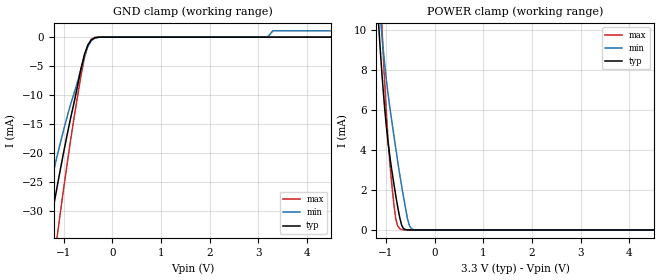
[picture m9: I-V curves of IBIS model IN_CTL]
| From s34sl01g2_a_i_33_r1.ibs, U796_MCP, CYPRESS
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|Driver/receiver models for NAND component of MCP
|   Model IN_CTL
[Model]  IN_CTL
Model_type Input
Vinl =   0.6600V | Vinl = Vio*0.3
Vinh =   2.6400V | Vinh = Vio*0.8
C_comp   3.14pF   2.83pF   4.09pF
[Temperature Range]   25.0000   85.0000   -40.0000
[Pullup Reference]   3.3000V   2.7000V   3.6000V
[Pulldown Reference]   0.0V   0.0V   0.0V
[POWER Clamp Reference]   3.3000V   2.7000V   3.6000V
[GND Clamp Reference]   0.0V   0.0V   0.0V
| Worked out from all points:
|   GND clamp passes 1 mA (typ) near -0.47 V on its own axis
|   POWER clamp passes 1 mA (typ) near -0.75 V on its own axis
[GND_clamp]
|Voltage   I(typ)   I(min)   I(max)
-3.3V     -993.2mA   -397.9mA   -1.959A
-1.48V    -42.63mA   -33.34mA   -57.88mA
-1.34V    -35.68mA   -28.07mA   -48.21mA
-1.27V    -32.3mA    -25.5mA    -43.51mA
-1.13V    -25.77mA   -20.52mA   -34.37mA
-780mV    -11.16mA   -9.617mA   -13.71mA
-570mV    -2.965mA   -3.308mA   -3.505mA
-500mV    -1.356mA   -1.606mA   -1.413mA
-360mV    -117uA     -187.5uA   -58.29uA
3.14V     756.3pA    21.25uA    371.5pA
3.3V      808.9pA    1.086mA    399pA
6.6V      808.9pA    1.086mA    399pA
[POWER_clamp]
|Voltage   I(typ)   I(min)   I(max)
-3.28V    954.7mA    449.2mA    1.77A
-1.16V    10.56mA    11.89mA    14.41mA
-1.12V    9.036mA    10.68mA    12.1mA
-1.08V    7.645mA    9.57mA     9.906mA
-1V       5.324mA    7.642mA    6.093mA
-960mV    4.398mA    6.817mA    4.554mA
-880mV    2.947mA    5.402mA    2.224mA
-800mV    1.702mA    4.066mA    543.8uA
-680mV    237.8uA    2.197mA    22.81uA
-520mV    1.459uA    215.4uA    122.7nA
-400mV    29.81nA    6.336uA    1.481nA
6.6V      0A         0A         0A
